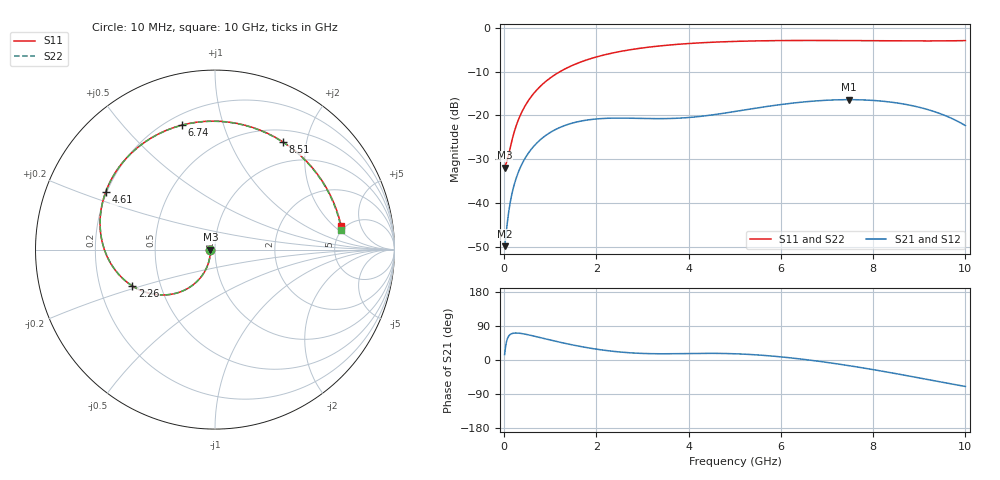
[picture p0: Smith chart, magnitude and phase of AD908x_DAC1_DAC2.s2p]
! Created Tue Jun 16 15:15:55 2020
# hz S ma R 50
! 2 Port Network Data from SP1.SP block
! freq  magS11  angS11  magS21  angS21  magS12  angS12  magS22  angS22
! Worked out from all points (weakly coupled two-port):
!   1000 points, 10 MHz to 10 GHz, reference 50 ohm
!   highest |S21| = -16.41 dB at 7.48 GHz (marker M1); lowest = -49.9 dB at 10 MHz (marker M2)
!   lowest |S11| = -32.0 dB at 10 MHz (marker M3), VSWR 1.05, Z = 47.5 - j0.0823 ohm
!   |S11| at or under -10 dB: start of sweep to 1.212 GHz
!   |S22| runs from -32.0 to -2.9 dB; largest |S21 - S12| = 0
!   S11 on the Smith chart (normalised r, x): 10 MHz: 0.95, -0.00; 2.26 GHz: 0.34, -0.19; 4.61 GHz: 0.20, +0.24; 6.74 GHz: 0.26, +0.74; 8.51 GHz: 0.66, +1.61; 10 GHz: 4.59, +2.51
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1e7  0.02519 -178.0  0.003197 14.4  0.003197 14.4  0.02511 -177.9
6e7  0.02976 -155.0  0.005392 52.5  0.005392 52.5  0.0296 -154.9
1.3e8  0.04236 -130.8  0.009982 67.2  0.009982 67.2  0.04239 -130.6
2.1e8  0.06237 -119.8  0.01556 70.9  0.01556 70.9  0.06255 -119.8
3.3e8  0.09465 -115.1  0.02393 70.7  0.02393 70.7  0.09499 -115.1
4.9e8  0.1379 -115.2  0.03471 67.3  0.03471 67.3  0.1385 -115.3
7.1e8  0.1959 -118.8  0.04839 61.2  0.04839 61.2  0.1966 -118.9
9.8e8  0.2629 -124.9  0.06282 53.4  0.06282 53.4  0.2639 -125.0
1.68e9  0.4106 -142.3  0.08632 35.1  0.08632 35.1  0.4118 -142.5
2.26e9  0.5036 -156.3  0.09269 24.3  0.09269 24.3  0.5048 -156.6
3.34e9  0.619 179.3  0.0917 16.4  0.0917 16.4  0.6198 178.9
3.97e9  0.6604 165.8  0.09418 17.1  0.09418 17.1  0.661 165.4
4.61e9  0.6885 152.3  0.1028 17.5  0.1028 17.5  0.6888 151.8
5.01e9  0.7004 143.8  0.1108 16.4  0.1108 16.4  0.7005 143.2
5.81e9  0.714 126.4  0.1288 10.4  0.1288 10.4  0.7137 125.7
6.67e9  0.7178 106.6  0.145 -1.0  0.145 -1.0  0.717 105.8
6.74e9  0.7177 105.0  0.146 -2.1  0.146 -2.1  0.7169 104.1
7.48e9  0.715 86.4  0.1511 -15.0  0.1511 -15.0  0.7138 85.4
8.34e9  0.7102 62.8  0.1426 -32.6  0.1426 -32.6  0.7086 61.5
8.51e9  0.7095 57.8  0.1388 -36.3  0.1388 -36.3  0.7078 56.5
9.32e9  0.7091 32.9  0.1107 -54.7  0.1107 -54.7  0.7073 31.3
1e10  0.7148 10.8  0.07637 -69.8  0.07637 -69.8  0.713 8.9
